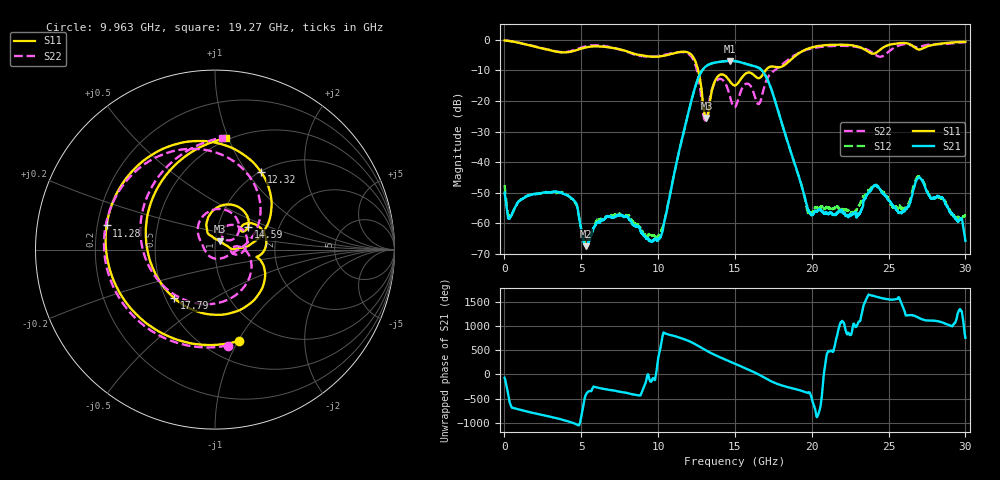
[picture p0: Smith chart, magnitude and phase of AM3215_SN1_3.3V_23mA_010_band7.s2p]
!Agilent Technologies,E8364B,MY43040894,A.07.50.67
!Agilent E8364B: A.07.50.67
!Date: Tuesday, May 25, 2021 15:17:29
!Correction: S11(Full 2 Port(1,2))
!S21(Full 2 Port(1,2))
!S12(Full 2 Port(1,2))
!S22(Full 2 Port(1,2))
!S2P File: Measurements: S11, S21, S12, S22:
# Hz S  dB  R 50
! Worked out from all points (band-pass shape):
!   6401 points, 10 MHz to 30 GHz, reference 50 ohm
!   highest |S21| = -6.93 dB at 14.7 GHz (marker M1); lowest = -67.4 dB at 5.286 GHz (marker M2)
!   |S21| within 3 dB of the highest: 12.89 GHz to 16.73 GHz (3.844 GHz wide, 26 % of centre)
!   lowest |S11| = -25.6 dB at 13.14 GHz (marker M3), VSWR 1.11, Z = 52.5 + j4.8 ohm
!   |S11| at or under -10 dB: 12.61 GHz to 17 GHz (4.392 GHz wide, 29.7 % of centre)
!   |S22| runs from -26.4 to -0.3 dB; largest |S21 - S12| = 0.0074
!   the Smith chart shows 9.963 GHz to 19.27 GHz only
!   S11 on the Smith chart (normalised r, x): 9.963 GHz: 0.71, -1.00; 11.28 GHz: 0.24, +0.10; 12.32 GHz: 1.01, +1.17; 14.59 GHz: 1.39, +0.37; 17.79 GHz: 0.55, -0.34; 19.27 GHz: 0.48, +0.98
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1e7  -0.27 -6.4  -49.85 -67.3  -47.51 108.6  -0.28 -6.5
9.331297e8  -1.04 -84.2  -52.77 -0.4  -52.71 2.2  -0.99 -84.2
2.006209e9  -2.34 -165.6  -50.39 -83.2  -50.41 -84.8  -2.24 -164.5
3.477594e9  -4.00 79.2  -49.68 171.8  -49.85 170.2  -3.94 83.6
5.009895e9  -2.93 -77.5  -62.52 -133.2  -62.03 155.6  -2.58 -74.0
5.286366e9  -2.57 -102.7  -67.40 -59.3  -65.55 143.1  -2.19 -100.1
6.265727e9  -2.22 -178.3  -59.09 72.8  -58.48 67.7  -1.94 -177.5
7.502814e9  -3.17 104.0  -57.16 4.9  -56.82 8.3  -3.22 101.8
9.962931e9  -5.58 -75.6  -65.64 -122.3  -64.39 66.3  -5.37 -82.5
1.000979e10  -5.56 -79.8  -65.30 -21.5  -64.10 94.7  -5.33 -86.3
1.127968e10  -4.17 167.4  -38.27 50.5  -38.46 51.5  -4.13 172.3
1.231527e10  -5.97 59.5  -17.13 -78.8  -17.12 -78.0  -6.80 66.4
1.314468e10  -25.56 59.9  -8.58 130.1  -8.62 130.3  -26.06 -151.0
1.458795e10  -13.01 34.6  -6.95 -82.4  -6.93 -82.0  -16.95 32.0
1.469573e10  -13.75 32.3  -6.93 -97.2  -6.93 -96.9  -18.89 29.8
1.5005e10  -14.94 36.5  -7.03 -139.8  -7.03 -139.5  -22.00 54.5
1.779313e10  -9.03 -130.4  -23.00 161.3  -22.97 161.0  -9.26 -138.6
1.927389e10  -4.10 84.5  -46.53 30.0  -46.45 31.0  -4.09 86.6
2.00049e10  -2.52 45.4  -57.07 -127.6  -56.70 168.7  -2.86 48.4
2.500479e10  -1.75 -55.8  -52.48 108.6  -52.33 104.7  -3.92 -54.3
2.704317e10  -3.20 -87.5  -45.06 75.7  -44.86 72.0  -2.30 -87.7
3e10  -0.72 -116.6  -65.68 35.4  -57.08 34.7  -0.83 -118.4
